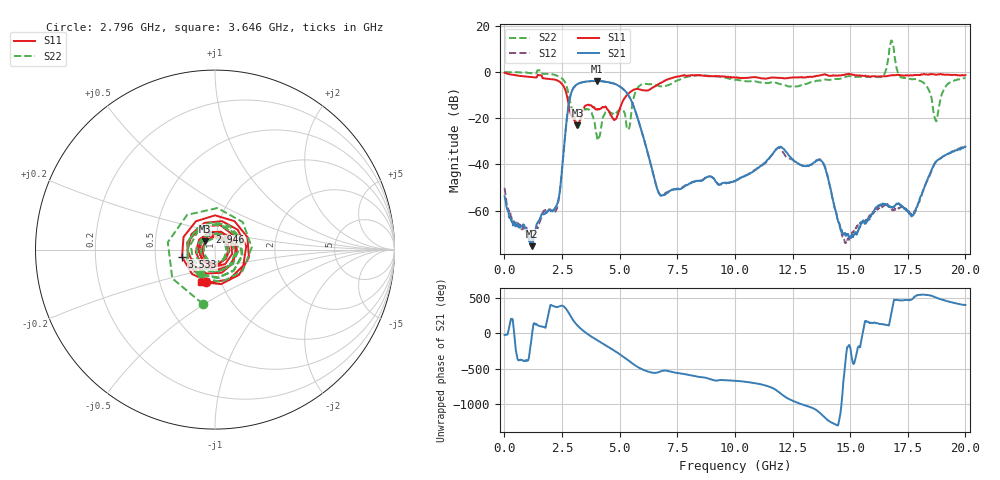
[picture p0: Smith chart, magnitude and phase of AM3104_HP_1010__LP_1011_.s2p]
!Created with skrf (http://scikit-rf.org).
# Hz S RI R 50.0
!freq ReS11 ImS11 ReS21 ImS21 ReS12 ImS12 ReS22 ImS22
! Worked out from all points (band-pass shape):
!   1601 points, 10 MHz to 20 GHz, reference 50 ohm
!   highest |S21| = -3.87 dB at 4.008 GHz (marker M1); lowest = -75.4 dB at 1.197 GHz (marker M2)
!   |S21| within 3 dB of the highest: 2.999 GHz to 5.093 GHz (2.094 GHz wide, 51.7 % of centre)
!   lowest |S11| = -23.0 dB at 3.171 GHz (marker M3), VSWR 1.15, Z = 44.7 + j4.12 ohm
!   |S11| at or under -10 dB: 2.706 GHz to 5.311 GHz (2.606 GHz wide, 65 % of centre)
!   |S22| runs from -29.6 to 13.6 dB; largest |S21 - S12| = 0.053
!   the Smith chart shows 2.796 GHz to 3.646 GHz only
!   S11 on the Smith chart (normalised r, x): 2.796 GHz: 0.85, -0.32; 2.946 GHz: 0.92, +0.18; 3.533 GHz: 0.69, -0.06; 3.646 GHz: 0.80, -0.30
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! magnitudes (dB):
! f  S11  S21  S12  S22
! 10 MHz  -0.4  -53.8  -50.2  -0.1
! 1.197 GHz  -2.2  -75.4  -74.1  -0.6
! 2.296 GHz  -3.7  -57.0  -58.6  -1.7
! 2.796 GHz  -14.6  -13.7  -13.7  -10.2
! 2.946 GHz  -19.8  -7.8  -7.9  -16.4
! 3.171 GHz  -23.0  -5.2  -5.3  -23.9
! 3.346 GHz  -18.8  -4.5  -4.6  -19.6
! 3.533 GHz  -14.5  -4.2  -4.3  -15.9
! 3.646 GHz  -14.1  -4.1  -4.2  -16.1
! 4.008 GHz  -16.2  -3.9  -3.9  -27.5
! 5.42 GHz  -9.0  -10.7  -10.8  -24.1
! 5.795 GHz  -7.3  -20.4  -20.4  -6.7
! 6.682 GHz  -5.3  -52.1  -52.0  -6.0
! 10.01 GHz  -2.5  -47.4  -47.1  -3.4
! 11.93 GHz  -2.5  -32.4  -32.8  -5.2
! 13.34 GHz  -2.1  -40.0  -39.9  -4.4
! 13.87 GHz  -1.1  -40.3  -39.9  -3.4
! 14.78 GHz  -1.2  -69.7  -73.7  -2.3
! 16.68 GHz  -1.6  -58.3  -58.3  7.2
! 17.74 GHz  -1.4  -62.0  -61.4  -3.1
! 18.71 GHz  -1.2  -38.9  -39.2  -21.1
! 20 GHz  -1.4  -32.4  -32.0  -2.6
